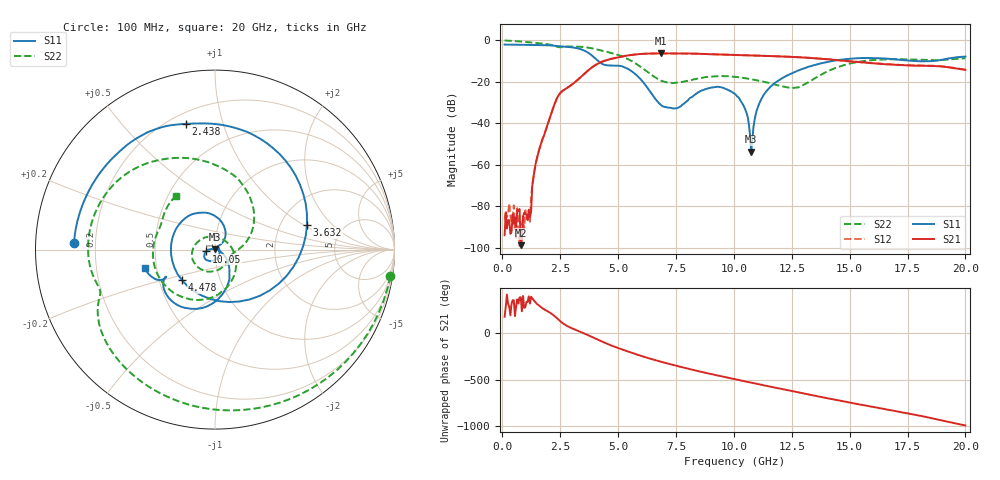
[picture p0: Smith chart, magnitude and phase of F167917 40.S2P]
!  2-Port S-parameters saved by WinCal
! VAR MeasName=S-Parameters (CALIBRATED_DATA) read from VNA (N5242A)
! VAR MeasDate=2016-11-22 9:01:44
! VAR NAME=F167917 40
! VAR FILENAME=F167917 40.S2P
! VAR DATE=2016-11-22 9:01:44
! VAR PHYS_PORTS=1,2
# Hz S DB R 50
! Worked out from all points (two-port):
!   401 points, 100 MHz to 20 GHz, reference 50 ohm
!   highest |S21| = -6.32 dB at 6.866 GHz (marker M1); lowest = -98.7 dB at 796.5 MHz (marker M2)
!   |S21| within 3 dB of the highest: 4.576 GHz to 14.21 GHz (9.638 GHz wide, 103 % of centre)
!   lowest |S11| = -53.6 dB at 10.75 GHz (marker M3), VSWR 1.00, Z = 49.9 + j0.2 ohm
!   |S11| at or under -10 dB: 4.14 GHz to 14.24 GHz (10.1 GHz wide, 110 % of centre); 17.82 GHz to 18.59 GHz (767.3 MHz wide, 4.22 % of centre)
!   |S22| runs from -23.0 to -0.1 dB; largest |S21 - S12| = 0.0058
!   S11 on the Smith chart (normalised r, x): 100 MHz: 0.12, +0.02; 2.438 GHz: 0.26, +0.76; 3.632 GHz: 2.80, +1.08; 4.478 GHz: 0.66, -0.24; 10.05 GHz: 0.91, -0.02; 20 GHz: 0.43, -0.11
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1e8  -2.09 177.3  -93.84 176.0  -86.39 129.7  -0.10 -8.7
7.965e8  -2.19 158.8  -98.67 25.7  -88.93 -75.2  -0.62 -63.3
1.14475e9  -2.25 149.1  -81.57 36.5  -81.86 -26.9  -0.96 -87.6
1.54275e9  -2.34 137.2  -54.78 -53.9  -54.70 -53.7  -1.38 -112.8
2.43825e9  -2.86 103.1  -26.40 143.1  -26.39 142.8  -3.31 -159.2
3.43325e9  -4.49 37.5  -17.28 8.0  -17.29 8.1  -3.20 158.0
3.63225e9  -5.50 15.1  -15.26 -13.3  -15.26 -13.2  -3.45 147.9
4.08e9  -9.41 -55.0  -11.56 -64.8  -11.52 -64.7  -4.41 125.6
4.478e9  -12.02 -136.9  -9.69 -108.8  -9.63 -109.0  -5.47 106.8
5.473e9  -14.08 95.2  -7.22 158.9  -7.23 158.6  -9.34 54.0
6.7665e9  -30.31 46.2  -6.33 59.0  -6.34 59.0  -18.98 -6.1
6.866e9  -31.29 48.4  -6.32 52.3  -6.34 52.2  -19.49 -9.3
8.657e9  -23.99 -100.6  -6.57 -59.0  -6.57 -59.0  -17.97 -103.1
1.005e10  -25.88 -168.1  -7.05 -135.0  -7.06 -134.9  -17.65 -167.3
1.049775e10  -33.43 172.5  -7.22 -158.4  -7.22 -158.4  -18.28 177.0
1.07465e10  -53.64 105.5  -7.32 -171.3  -7.30 -171.2  -18.76 168.5
1.1045e10  -32.02 -16.6  -7.42 173.4  -7.40 173.4  -19.41 158.1
1.149275e10  -23.40 -33.7  -7.57 150.5  -7.55 150.6  -20.53 140.5
1.338325e10  -12.25 -78.6  -8.56 54.0  -8.51 54.3  -19.10 -11.8
1.467675e10  -9.28 -106.6  -9.80 -9.5  -9.73 -9.6  -12.26 -83.5
1.67165e10  -8.96 -143.4  -11.61 -104.1  -11.60 -104.4  -9.15 -156.7
2e10  -7.86 -165.1  -14.24 89.4  -14.15 88.8  -8.65 126.4
